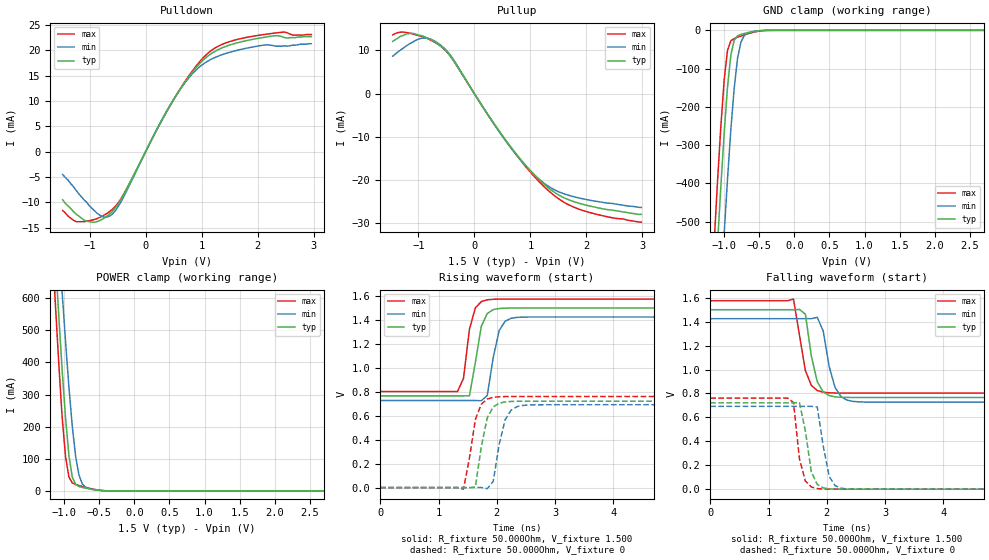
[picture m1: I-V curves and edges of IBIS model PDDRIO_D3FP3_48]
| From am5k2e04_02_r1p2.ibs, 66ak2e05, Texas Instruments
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|   Model PDDRIO_D3FP3_48
[Model] PDDRIO_D3FP3_48
Model_type   I/O
Polarity   Non-Inverting
Enable   Active-High
C_comp   3.236pF   3.174pF   3.318pF
C_comp_pullup   516.723fF   493.565fF   544.031fF
C_comp_pulldown 2.715pF   2.675pF   2.769pF
Vinh = 925.000mV
Vinl = 575.000mV
Vmeas = 750.000mV
Vref = 750.000mV
Rref = 50Ohms
Cref = 0pF
[Model Spec]
Vinh   925.000mV   888.000mV   963.000mV
Vinl   575.000mV   538.000mV   613.000mV
Vmeas   750.000mV   713.000mV   788.000mV
Vref   750.000mV   713.000mV   788.000mV
[Temperature Range]   25.000   125.000   -40.000
[Voltage Range]   1.500V   1.425V   1.575V
[GND Clamp Reference]   0.00V   0.00V   0.00V
|[C Comp Corner]
| variable   typ   min   max
|C_comp 3.236pF   3.318pF   3.174pF
|C_comp_pullup 516.723fF   544.031fF   493.565fF
|C_comp_pulldown 2.715pF   2.769pF   2.675pF
[Pulldown Reference]   0.00V   0.00V   0.00V
[POWER Clamp Reference]   1.500V   1.425V   1.575V
[Pullup Reference]   1.500V   1.425V   1.575V
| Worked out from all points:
|   slope of the pulldown table from 0 to 0.225 V, typ, clamps not added: 46.4 ohm
|   slope of the pullup table from 0 to 0.225 V, typ, clamps not added: 50 ohm
|   GND clamp passes 1 mA (typ) near -0.49 V on its own axis
|   POWER clamp passes 1 mA (typ) near -0.46 V on its own axis
|   rising waveform, R_fixture 50.000Ohm, V_fixture 1.500: 20-80 % time 156ps typ, 162ps min, 147ps max; typ from 0.766 V to 1.5 V
|   rising waveform, R_fixture 50.000Ohm, V_fixture 0: 20-80 % time 160ps typ, 170ps min, 171ps max; typ from 0 V to 0.722 V
|   falling waveform, R_fixture 50.000Ohm, V_fixture 1.500: 20-80 % time 165ps typ, 182ps min, 175ps max; typ from 1.5 V to 0.766 V
|   falling waveform, R_fixture 50.000Ohm, V_fixture 0: 20-80 % time 141ps typ, 150ps min, 133ps max; typ from 0.722 V to 0 V
[GND Clamp]
-1.48V    -1.918A    -2.181A    -1.764A
-1.145V   -723.4mA   -1.002A    -556.7mA
-1.098V   -563.3mA   -840.4mA   -399.2mA
-1.05V    -410.5mA   -683.3mA   -253.2mA
-1.002V   -269.5mA   -532mA     -130mA
-954.6mV  -149.1mA   -389.4mA   -52.57mA
-906.8mV  -64.77mA   -260.1mA   -27.53mA
-859.1mV  -26.06mA   -151.5mA   -21.41mA
-811.4mV  -14.61mA   -73.73mA   -17.98mA
-715.9mV  -8.245mA   -13.8mA    -12.04mA
-525mV    -1.646mA   -1.444mA   -2.745mA
2.959V    5.133nA    157.9nA    5.129nA
[Power Clamp]
-1.459V   2.052A     2.172A     2.008A
-1.173V   897.3mA    1.113A     766.5mA
-1.125V   714.9mA    943mA      572.9mA
-1.077V   539.1mA    776.9mA    390mA
-1.03V    373.7mA    616.2mA    227.4mA
-981.8mV  225.9mA    463.5mA    105.8mA
-934.1mV  109.7mA    322.9mA    43.29mA
-886.4mV  43.23mA    201.1mA    25.08mA
-838.6mV  20.27mA    107.7mA    20.03mA
-790.9mV  13.81mA    49.43mA    16.8mA
-647.7mV  6.613mA    6.926mA    8.545mA
2.98V     -9.151nA   -320.3nA   -14.09nA
[Pulldown]
-1.48V    -9.5mA     -4.5mA     -11.6mA
-1.241V   -12.3mA    -7.6mA     -13.8mA
-1.05V    -13.7mA    -10mA      -13.7mA
-859.1mV  -13.76mA   -12.2mA    -13.15mA
-668.2mV  -12.53mA   -12.84mA   -12.01mA
-381.8mV  -8.307mA   -8.695mA   -8.19mA
477.3mV   9.81mA     9.914mA    9.849mA
954.6mV   17.24mA    16.65mA    17.6mA
1.241V    19.81mA    18.59mA    20.46mA
1.67V     21.57mA    20.09mA    22.23mA
2.434V    22.7mA     20.8mA     23.56mA
2.959V    22.7mA     21.3mA     23.1mA
[Pullup]
-1.459V   12.1mA     8.686mA    13.63mA
-1.316V   13.3mA     10.13mA    14.24mA
-1.125V   14mA       11.77mA    13.91mA
-886.4mV  13.16mA    12.9mA     13mA
-695.5mV  11.89mA    12.09mA    11.79mA
-409.1mV  8.358mA    8.567mA    8.344mA
211.4mV   -4.23mA    -4.334mA   -4.267mA
640.9mV   -12.14mA   -12.31mA   -12.3mA
1.214V    -20.59mA   -20.37mA   -21.1mA
1.5V      -23.38mA   -22.64mA   -24.26mA
1.834V    -25.19mA   -24mA      -26.53mA
2.98V     -27.9mA    -26.3mA    -29.7mA
[Ramp]
R_load=50.000Ohm
dV/dt_r   436.650mV/149.500ps  416.999mV/159.000ps  460.020mV/140.500ps
dV/dt_f   436.650mV/142.000ps  416.999mV/151.500ps  460.020mV/136.000ps
[Rising waveform]
R_fixture=50.000Ohm
V_fixture=1.500
V_fixture_min=1.425
V_fixture_max=1.575
0s        766mV      727.3mV    802.9mV
1.327ns   766mV      727.3mV    802.9mV
1.429ns   766.1mV    727.3mV    912.8mV
1.531ns   766.9mV    727.3mV    1.323V
1.633ns   1.046V     727.4mV    1.501V
1.735ns   1.348V     725.6mV    1.554V
1.837ns   1.454V     769.6mV    1.569V
2.042ns   1.496V     1.312V     1.575V
2.246ns   1.5V       1.414V     1.575V
10ns      1.5V       1.425V     1.575V
[Rising waveform]
R_fixture=50.000Ohm
V_fixture=0
0s        0V         2.363uV    0V
1.429ns   31.14uV    -4.072uV   -13.2mV
1.633ns   5.3mV      13.99uV    569.2mV
1.735ns   342.4mV    432.1uV    696.4mV
1.837ns   582.5mV    -8.968mV   739.9mV
1.939ns   673.8mV    51.21mV    754.2mV
2.042ns   705.3mV    362mV      758.9mV
2.144ns   715.9mV    566.3mV    760.4mV
2.45ns    721.2mV    686.6mV    761.3mV
10ns      721.5mV    692.3mV    761.3mV
[Falling waveform]
R_fixture=50.000Ohm
V_fixture=1.500
V_fixture_min=1.425
V_fixture_max=1.575
0s        1.5V       1.425V     1.575V
1.429ns   1.5V       1.425V     1.589V
1.633ns   1.463V     1.425V     990.8mV
1.735ns   1.115V     1.425V     867.7mV
1.837ns   898.4mV    1.436V     824.7mV
1.939ns   813.4mV    1.322V     810.3mV
2.042ns   782.2mV    1.024V     805.5mV
2.144ns   771.6mV    849mV      803.8mV
2.45ns    766.3mV    733.6mV    803mV
10ns      766mV      727.3mV    802.9mV
[Falling waveform]
R_fixture=50.000Ohm
V_fixture=0
0s        721.5mV    692.3mV    761.3mV
1.327ns   721.5mV    692.3mV    761.3mV
1.429ns   721.5mV    692.3mV    723.7mV
1.531ns   723mV      692.3mV    254.3mV
1.633ns   486.7mV    692.3mV    68.26mV
1.735ns   144.6mV    692.3mV    18.21mV
1.837ns   39.48mV    687.5mV    4.755mV
2.042ns   2.903mV    106.4mV    318uV
2.246ns   206.9uV    8.191mV    19.2uV
10ns      0V         2.36uV     0V
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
